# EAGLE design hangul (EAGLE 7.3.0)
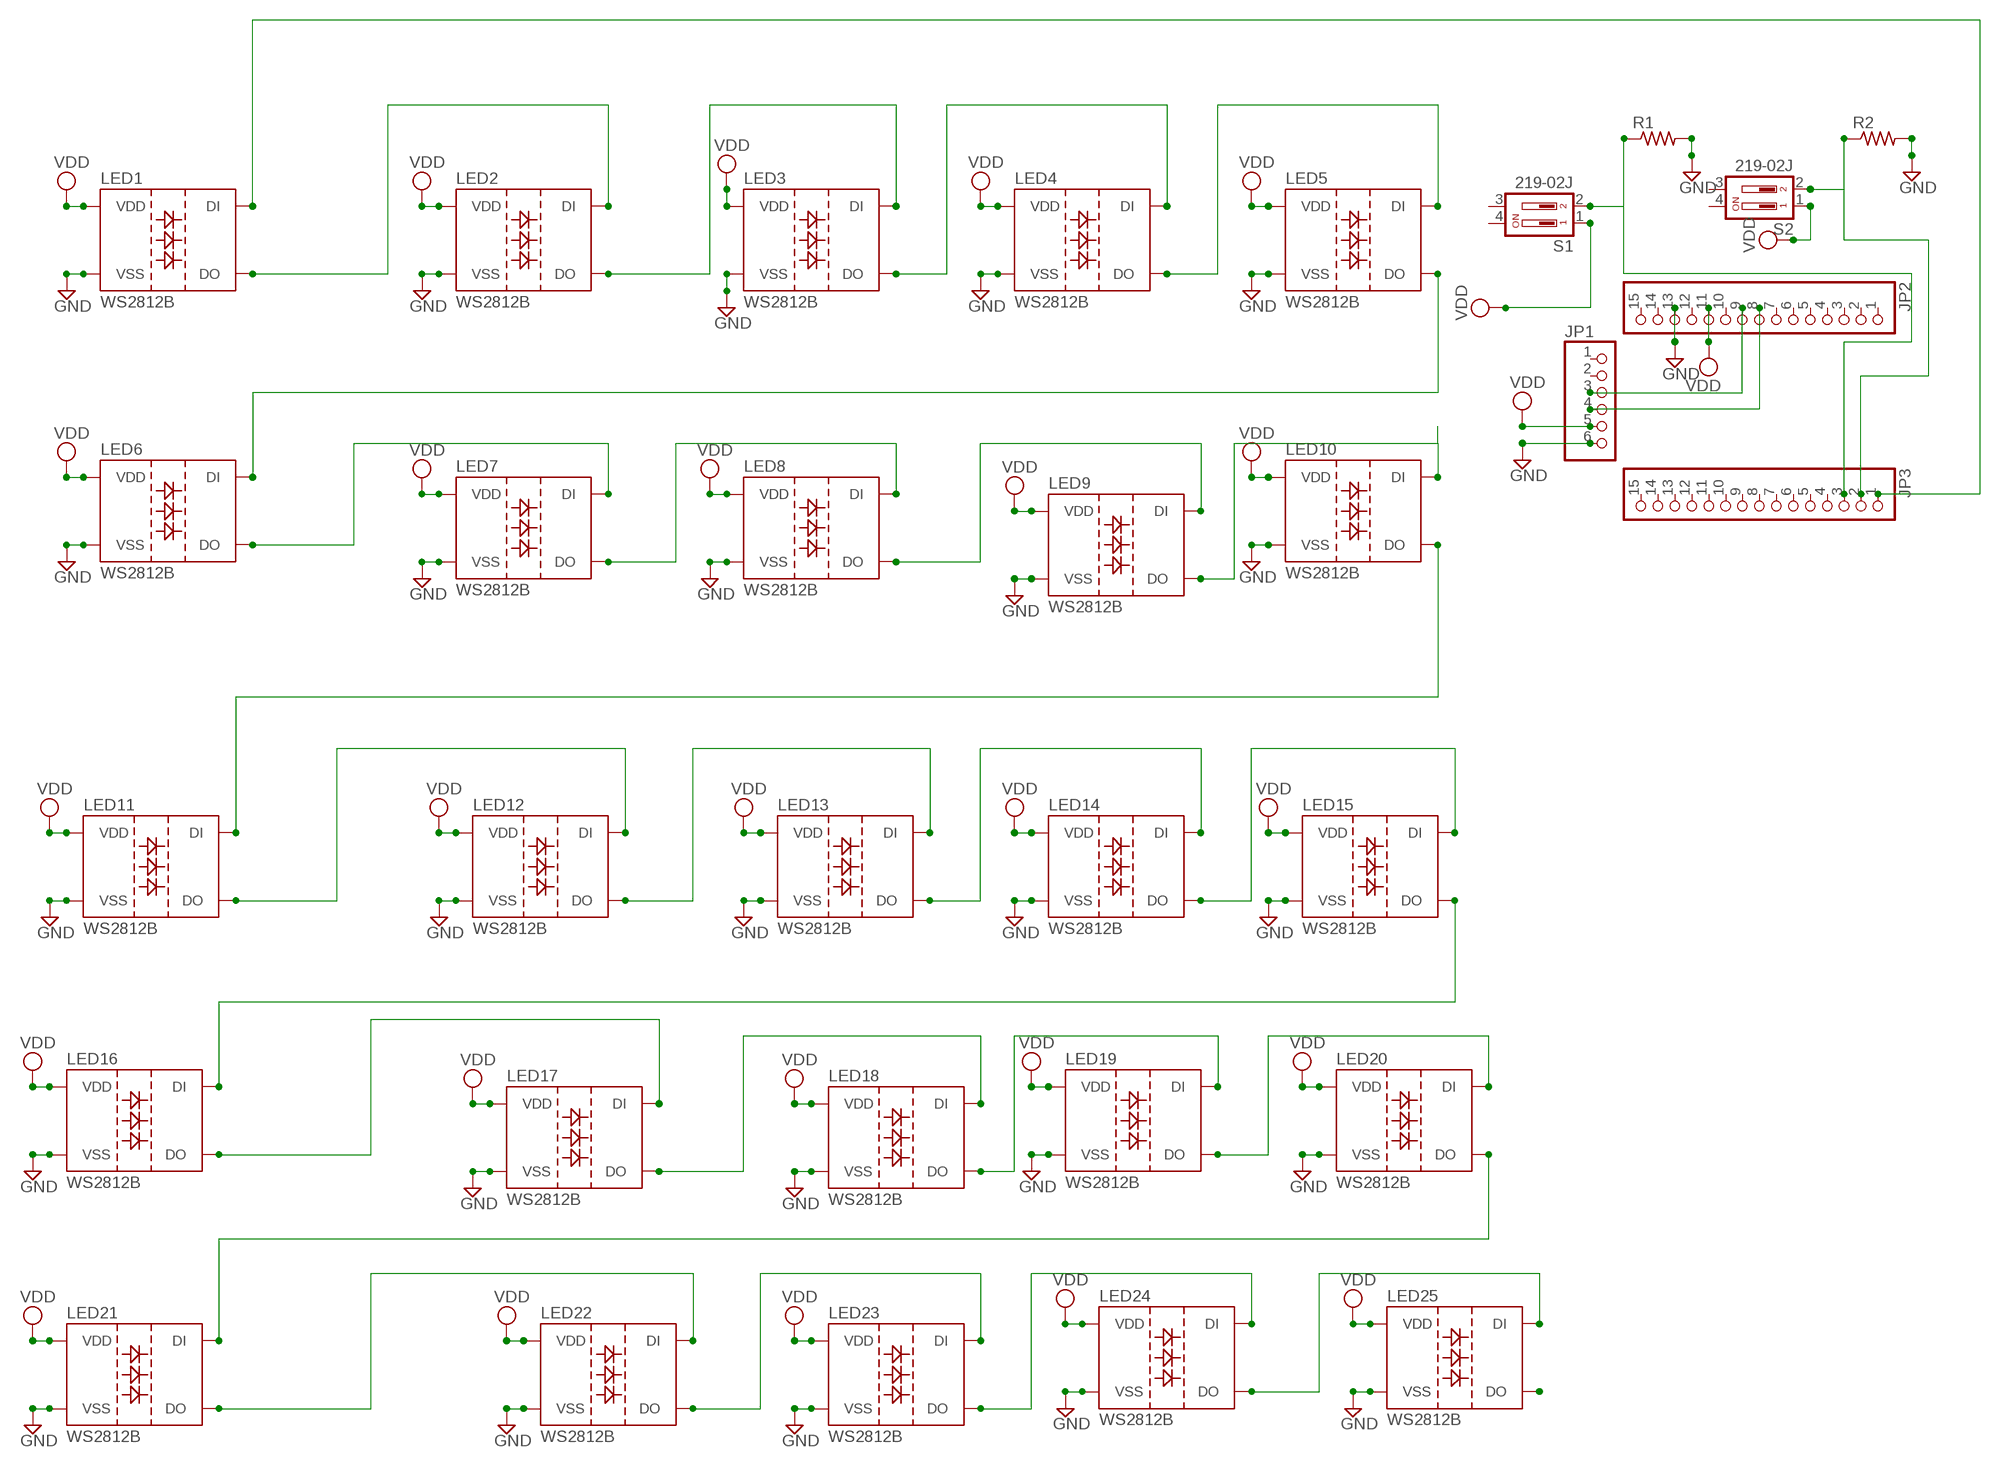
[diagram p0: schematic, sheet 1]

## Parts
JP1  PINHD-1X6  [1X06]
JP2  PINHD-1X15  [1X15]
JP3  PINHD-1X15  [1X15]
LED1  WS2812B  [WS2812B]
LED2  WS2812B  [WS2812B]
LED3  WS2812B  [WS2812B]
LED4  WS2812B  [WS2812B]
LED5  WS2812B  [WS2812B]
LED6  WS2812B  [WS2812B]
LED7  WS2812B  [WS2812B]
LED8  WS2812B  [WS2812B]
LED9  WS2812B  [WS2812B]
LED10  WS2812B  [WS2812B]
LED11  WS2812B  [WS2812B]
LED12  WS2812B  [WS2812B]
LED13  WS2812B  [WS2812B]
LED14  WS2812B  [WS2812B]
LED15  WS2812B  [WS2812B]
LED16  WS2812B  [WS2812B]
LED17  WS2812B  [WS2812B]
LED18  WS2812B  [WS2812B]
LED19  WS2812B  [WS2812B]
LED20  WS2812B  [WS2812B]
LED21  WS2812B  [WS2812B]
LED22  WS2812B  [WS2812B]
LED23  WS2812B  [WS2812B]
LED24  WS2812B  [WS2812B]
LED25  WS2812B  [WS2812B]
R1  R-US_0207/10  [0207/10]
R2  R-US_0207/10  [0207/10]
S1  219-02J  [CTS-219-02J]
S2  219-02J  [CTS-219-02J]

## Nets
GND: JP1.6 JP2.13 LED1.3(VSS) LED2.3(VSS) LED3.3(VSS) LED4.3(VSS) LED5.3(VSS) LED6.3(VSS) LED7.3(VSS) LED8.3(VSS) LED9.3(VSS) LED10.3(VSS) LED11.3(VSS) LED12.3(VSS) LED13.3(VSS) LED14.3(VSS) LED15.3(VSS) LED16.3(VSS) LED17.3(VSS) LED18.3(VSS) LED19.3(VSS) LED20.3(VSS) LED21.3(VSS) LED22.3(VSS) LED23.3(VSS) LED24.3(VSS) LED25.3(VSS) R1.2 R2.2
N$1: JP3.2 R2.1 S2.2
N$2: JP3.3 R1.1 S1.2
N$3: JP3.1 LED1.4(DI)
N$4: LED1.2(DO) LED2.4(DI)
N$7: JP1.3 JP2.9
N$8: LED2.2(DO) LED3.4(DI)
N$12: LED3.2(DO) LED4.4(DI)
N$16: LED4.2(DO) LED5.4(DI)
N$20: LED5.2(DO) LED6.4(DI)
N$21: JP1.4 JP2.8
N$22: LED10.2(DO) LED11.4(DI)
N$26: LED9.2(DO) LED10.4(DI)
N$30: LED8.2(DO) LED9.4(DI)
N$34: LED7.2(DO) LED8.4(DI)
N$38: LED6.2(DO) LED7.4(DI)
N$44: LED11.2(DO) LED12.4(DI)
N$48: LED12.2(DO) LED13.4(DI)
N$52: LED13.2(DO) LED14.4(DI)
N$56: LED14.2(DO) LED15.4(DI)
N$60: LED15.2(DO) LED16.4(DI)
N$62: LED20.2(DO) LED21.4(DI)
N$66: LED19.2(DO) LED20.4(DI)
N$70: LED18.2(DO) LED19.4(DI)
N$74: LED17.2(DO) LED18.4(DI)
N$78: LED16.2(DO) LED17.4(DI)
N$84: LED21.2(DO) LED22.4(DI)
N$88: LED22.2(DO) LED23.4(DI)
N$92: LED23.2(DO) LED24.4(DI)
N$96: LED24.2(DO) LED25.4(DI)
N$100: LED25.2(DO)
VDD: JP1.5 JP2.11 LED1.1(VDD) LED2.1(VDD) LED3.1(VDD) LED4.1(VDD) LED5.1(VDD) LED6.1(VDD) LED7.1(VDD) LED8.1(VDD) LED9.1(VDD) LED10.1(VDD) LED11.1(VDD) LED12.1(VDD) LED13.1(VDD) LED14.1(VDD) LED15.1(VDD) LED16.1(VDD) LED17.1(VDD) LED18.1(VDD) LED19.1(VDD) LED20.1(VDD) LED21.1(VDD) LED22.1(VDD) LED23.1(VDD) LED24.1(VDD) LED25.1(VDD) S1.1 S2.1
Unconnected: JP1.1 JP1.2 JP2.1 JP2.2 JP2.3 JP2.4 JP2.5 JP2.6 JP2.7 JP2.10 JP2.12 JP2.14 JP2.15 JP3.4 JP3.5 JP3.6 JP3.7 JP3.8 JP3.9 JP3.10 JP3.11 JP3.12 JP3.13 JP3.14 JP3.15 S1.3 S1.4 S2.3 S2.4

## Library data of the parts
JP1 = adafruit:PINHD-1X6: PIN HEADER
JP2 JP3 = adafruit:PINHD-1X15: PIN HEADER
LED1-LED25 = WS2812:WS2812B
R1 R2 = adafruit:R-US_: RESISTOR, American symbol
S1 S2 = switch-dil:219-02*: Surface Mount DIP Switch Series 219 SMT CTS Electronic Components Sourc: www.ctscorp.com; OC_FARNELL: unknown; OC_NEWARK: unknown

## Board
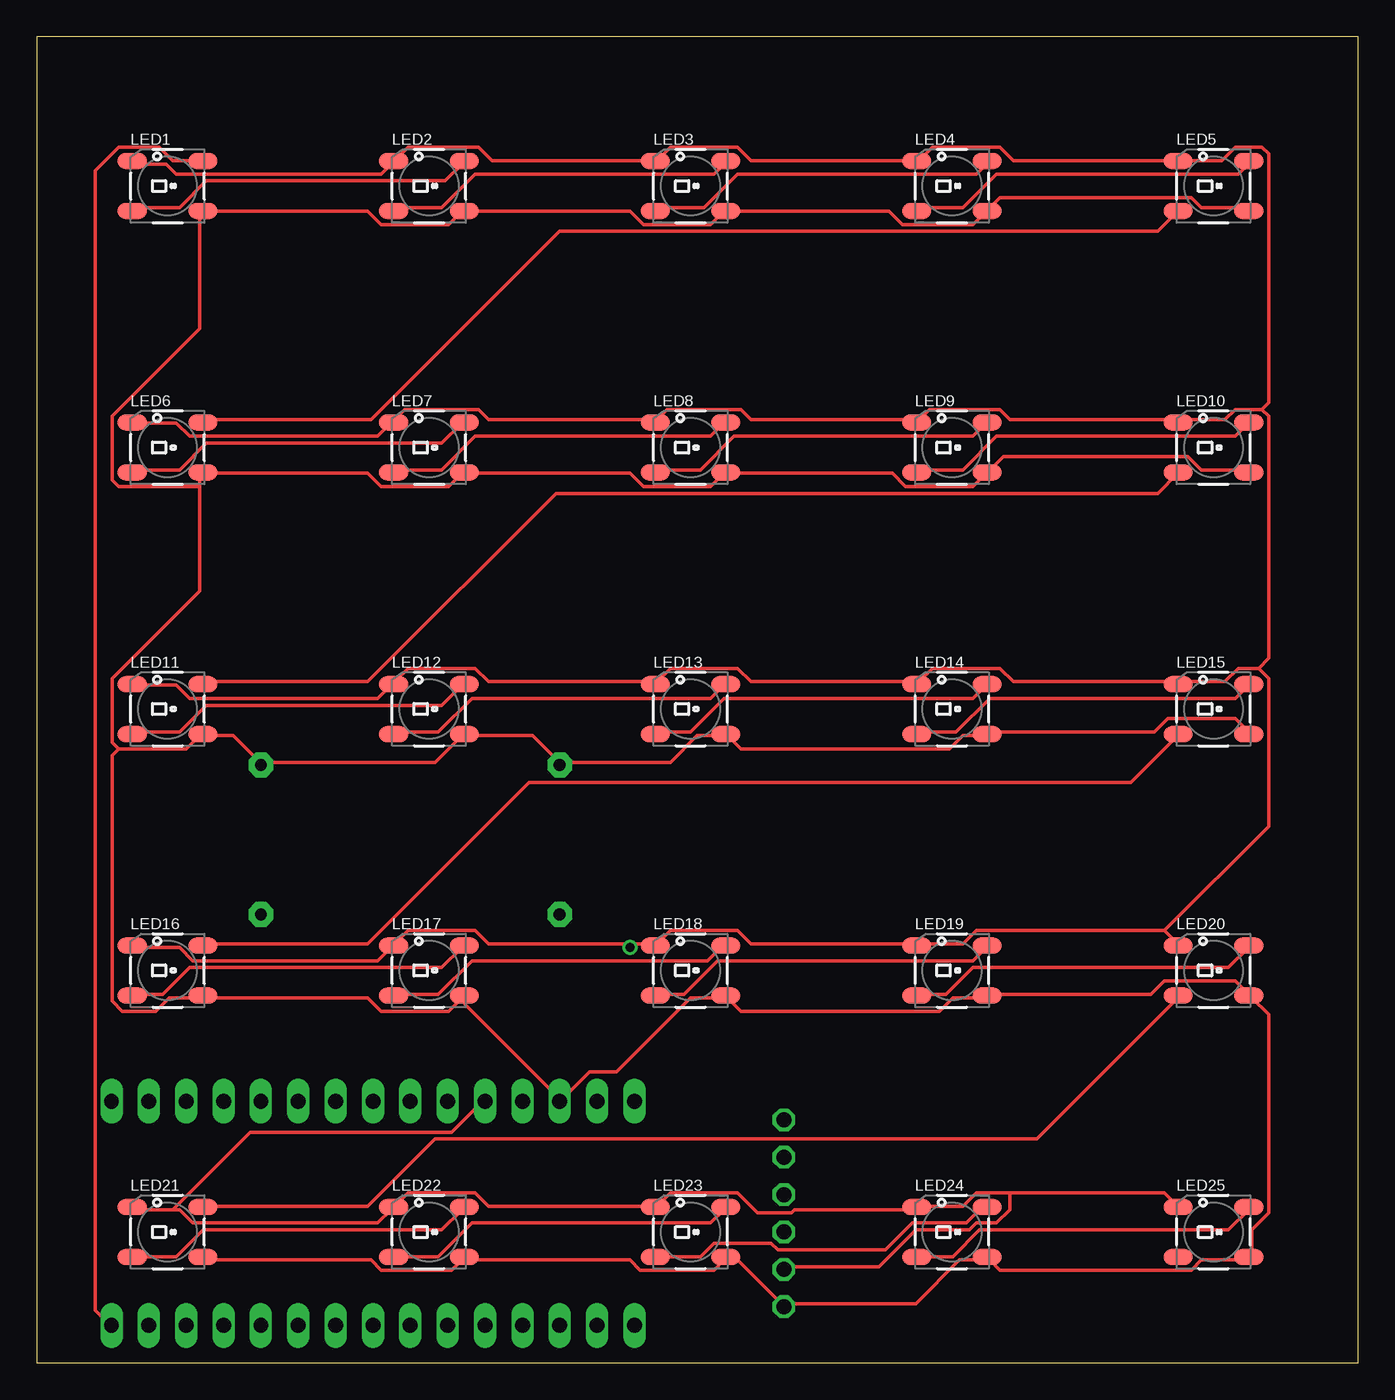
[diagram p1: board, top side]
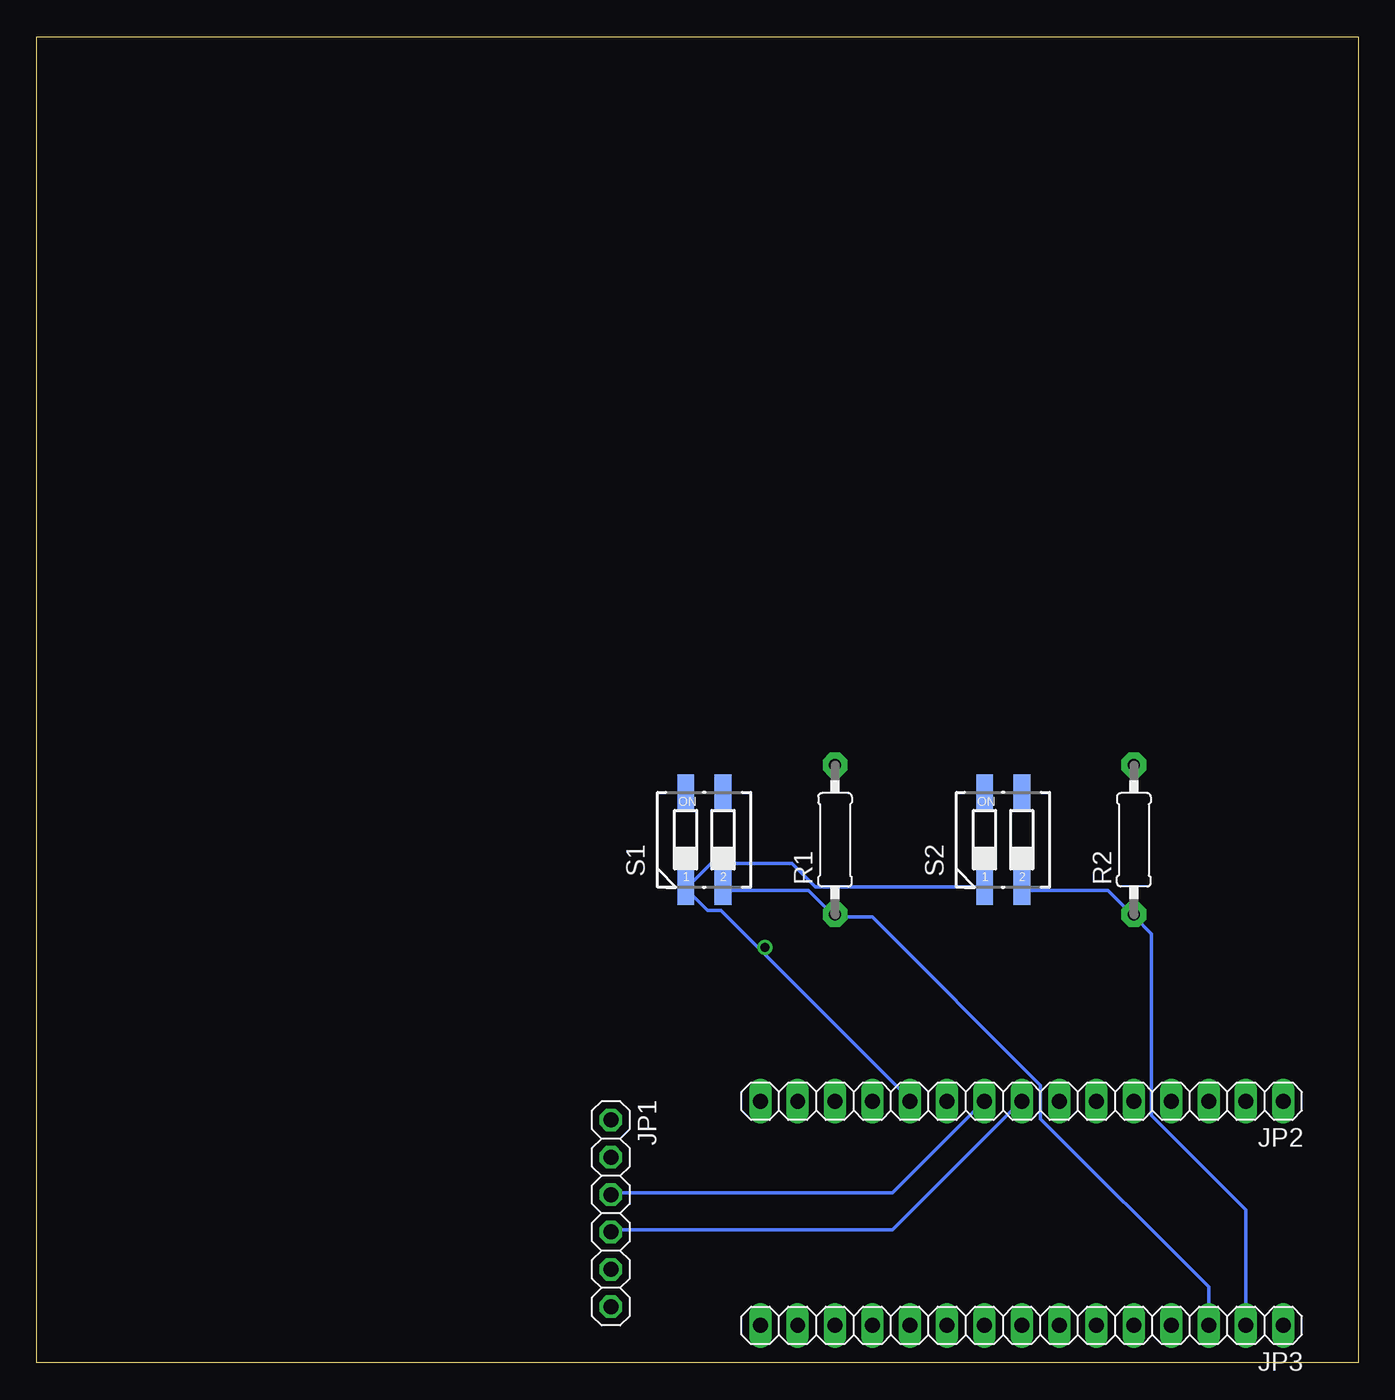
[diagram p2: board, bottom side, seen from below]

Size 89.84 x 90.16 mm. Coordinates in mm from the lower left corner, seen from the top.
Outline: 0,0 89.84,0 89.84,90.16 0,90.16 0,0
Copper layers (1*16): Top 0.035mm / dielectric 1.5mm / Bottom 0.035mm
Design rules "default": minimum track width 10mil, minimum drill 24mil, track to track 8mil, track to pad 8mil, pad to pad 8mil, via to via 8mil, smd to smd 8mil, copper to edge 40mil, drill to drill 8mil, minimum pad ring 10mil, minimum via ring 8mil, stop-mask expansion 4mil, vias tented up to drill 0mil, thermal gap 10mil

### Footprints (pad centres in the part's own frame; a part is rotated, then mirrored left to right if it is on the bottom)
1X06 = drill 1.016 octagon: 1 -6.35,0; 2 -3.81,0; 3 -1.27,0; 4 1.27,0; 5 3.81,0; 6 6.35,0
1X15 = drill 1.016 long: 1 -17.78,0; 2 -15.24,0; 3 -12.7,0; 4 -10.16,0; 5 -7.62,0; 6 -5.08,0; 7 -2.54,0; 8 0,0; 9 2.54,0; 10 5.08,0; 11 7.62,0; 12 10.16,0; 13 12.7,0; 14 15.24,0; 15 17.78,0
WS2812B = smd 2 x 1.1: 1 -2.4,1.7; 2 -2.4,-1.7; 3 2.4,-1.7; 4 2.4,1.7
0207/10 = drill 0.813 pad 1.676 octagon: 1 -5.08,0; 2 5.08,0
CTS-219-02J = smd 1.13 x 2.44: 1 -1.27,-3.215; 2 1.27,-3.215; 3 1.27,3.215; 4 -1.27,3.215

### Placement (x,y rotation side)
JP1  50.8,10.16 270 bottom
JP2  22.86,17.78 180 bottom
JP3  22.86,2.54 180 bottom
LED1  8.89,80.01 0 top
LED2  26.67,80.01 0 top
LED3  44.45,80.01 0 top
LED4  62.23,80.01 0 top
LED5  80.01,80.01 0 top
LED6  8.89,62.23 0 top
LED7  26.67,62.23 0 top
LED8  44.45,62.23 0 top
LED9  62.23,62.23 0 top
LED10  80.01,62.23 0 top
LED11  8.89,44.45 0 top
LED12  26.67,44.45 0 top
LED13  44.45,44.45 0 top
LED14  62.23,44.45 0 top
LED15  80.01,44.45 0 top
LED16  8.89,26.67 0 top
LED17  26.67,26.67 0 top
LED18  44.45,26.67 0 top
LED19  62.23,26.67 0 top
LED20  80.01,26.67 0 top
LED21  8.89,8.89 0 top
LED22  26.67,8.89 0 top
LED23  44.45,8.89 0 top
LED24  62.23,8.89 0 top
LED25  80.01,8.89 0 top
R1  35.56,35.56 90 bottom
R2  15.24,35.56 90 bottom
S1  44.45,35.56 0 bottom
S2  24.13,35.56 0 bottom

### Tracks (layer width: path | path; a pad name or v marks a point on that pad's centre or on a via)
GND
  Top 0.254: LED21.3 11.3,6.98 22.73,6.98 23.42,6.3 28.22,6.3 28.91,6.98 LED22.3 29.13,6.98 40.33,6.98 41.02,6.3 46.05,6.3 46.74,6.98 LED23.3 46.96,6.98 47.65,6.98 50.62,4.01 JP1.6 50.85,4.01 59.77,4.01 62.74,6.98 64.57,6.98 LED24.3 64.8,6.98 65.48,6.3 78.51,6.3 79.2,6.98 82.4,6.98 LED25.3 82.63,7.21 82.63,9.04 83.77,10.18 83.77,23.67 82.63,24.82 LED20.3 82.4,25.04 81.48,25.96 76.68,25.96 75.77,25.04 64.8,25.04 LED19.3 64.57,24.82 62.28,24.82 61.37,23.9 47.88,23.9 46.96,24.82 LED18.3 46.74,24.82 44.45,24.82 39.42,19.79 37.59,19.79 35.76,17.96 JP2.13 35.53,17.96 29.13,24.36 29.13,24.82 LED17.3 28.91,24.82 27.99,23.9 23.42,23.9 22.5,24.82 11.3,24.82 LED16.3 11.07,24.82 9.02,24.82 8.1,23.9 5.82,23.9 5.13,24.59 5.13,41.28 5.59,41.73 | LED5.3 82.4,78.54 79.2,78.54 78.51,79.22 65.48,79.22 64.8,78.54 LED4.3 64.57,78.31 63.65,77.39 58.85,77.39 57.94,78.31 46.96,78.31 LED3.3 46.74,78.31 45.82,77.39 41.25,77.39 40.33,78.31 29.13,78.31 LED2.3 28.91,78.31 27.99,77.39 23.42,77.39 22.5,78.31 11.3,78.31 LED1.3 11.07,78.31 11.07,70.31 5.13,64.36 5.13,60.02 5.59,59.56 11.07,59.56 | LED10.3 82.4,60.71 79.2,60.71 78.28,61.62 65.71,61.62 64.8,60.71 LED9.3 64.57,60.48 63.65,59.56 59.08,59.56 58.17,60.48 46.96,60.48 LED8.3 46.74,60.48 45.82,59.56 41.25,59.56 40.33,60.48 29.13,60.48 LED7.3 28.91,60.48 27.99,59.56 23.42,59.56 22.5,60.48 11.3,60.48 LED6.3 11.07,60.48 11.07,59.56 | LED15.3 82.4,42.88 81.48,43.79 76.91,43.79 76,42.88 64.8,42.88 LED14.3 64.57,42.65 62.97,42.65 62.05,41.73 47.88,41.73 46.96,42.65 LED13.3 46.74,42.65 44.91,42.65 43.08,40.82 35.76,40.82 R1.2 35.53,40.82 33.71,42.65 29.13,42.65 LED12.3 28.91,42.65 27.08,40.82 15.42,40.82 R2.2 15.19,40.82 13.36,42.65 11.3,42.65 LED11.3 11.07,42.65 10.16,41.73 5.59,41.73
  Top 0.254: 11.07,59.56 11.07,52.48 5.13,46.53 5.13,42.19 5.59,41.73
N$1
  Bottom 0.254: S2.2 22.73,32.13 17.02,32.13 15.42,30.53 R2.1 15.19,30.3 14.05,29.16 14.05,16.82 7.64,10.41 7.64,2.64 JP3.2
N$2
  Bottom 0.254: S1.2 43.08,32.13 37.36,32.13 35.76,30.53 R1.1 35.53,30.3 33.02,30.3 21.59,18.87 21.59,16.59 10.16,5.16 JP3.3
N$3
  Top 0.254: LED1.4 11.07,81.74 9.25,81.74 8.33,82.65 5.59,82.65 3.99,81.05 3.99,3.56 4.9,2.64 JP3.1
N$4
  Top 0.254: LED1.2 6.5,78.54 9.7,78.54 11.53,80.37 27.76,80.37 28.91,81.51 LED2.4
N$7
  Bottom 0.254: JP1.3 50.62,11.56 31.65,11.56 25.48,17.73 JP2.9
N$8
  Top 0.254: LED2.2 24.33,78.54 27.53,78.54 29.82,80.82 46.05,80.82 46.74,81.51 LED3.4
N$12
  Top 0.254: LED3.2 42.16,78.54 45.36,78.54 47.65,80.82 63.88,80.82 64.57,81.51 LED4.4
N$16
  Top 0.254: LED4.2 59.99,78.54 62.97,78.54 65.25,80.82 81.71,80.82 82.4,81.51 LED5.4
N$20
  Top 0.254: LED6.4 11.3,64.14 22.73,64.14 35.53,76.94 76.23,76.94 77.6,78.31 LED5.2
N$21
  Bottom 0.254: JP1.4 50.62,9.04 31.65,9.04 22.96,17.73 JP2.8
N$22
  Top 0.254: LED11.4 11.3,46.3 22.5,46.3 35.31,59.11 76.23,59.11 77.6,60.48 LED10.2
N$26
  Top 0.254: LED9.2 59.99,60.71 62.97,60.71 65.25,62.99 81.48,62.99 82.4,63.91 LED10.4
N$30
  Top 0.254: LED8.2 42.16,60.71 45.14,60.71 47.42,62.99 63.65,62.99 64.57,63.91 LED9.4
N$34
  Top 0.254: LED7.2 24.33,60.71 27.53,60.71 29.82,62.99 45.82,62.99 46.74,63.91 LED8.4
N$38
  Top 0.254: LED6.2 6.5,60.71 9.7,60.71 11.53,62.54 27.53,62.54 28.91,63.91 LED7.4
N$44
  Top 0.254: LED11.2 6.5,42.88 9.7,42.88 11.53,44.7 27.53,44.7 28.91,46.08 LED12.4
N$48
  Top 0.254: LED12.2 24.33,42.88 27.3,42.88 29.59,45.16 45.82,45.16 46.74,46.08 LED13.4
N$52
  Top 0.254: LED13.2 42.16,42.88 44.45,42.88 46.74,45.16 63.65,45.16 64.57,46.08 LED14.4
N$56
  Top 0.254: LED14.2 59.99,42.88 62.51,42.88 64.8,45.16 81.48,45.16 82.4,46.08 LED15.4
N$60
  Top 0.254: LED16.4 11.3,28.47 22.5,28.47 33.48,39.45 74.4,39.45 77.6,42.65 LED15.2
N$62
  Top 0.254: LED21.4 11.3,10.64 22.5,10.64 27.08,15.21 68,15.21 77.6,24.82 LED20.2
N$66
  Top 0.254: LED19.2 59.99,25.04 61.82,25.04 63.65,26.87 81.03,26.87 82.4,28.25 LED20.4
N$70
  Top 0.254: LED18.2 42.16,25.04 43.99,25.04 46.28,27.33 63.65,27.33 64.57,28.25 LED19.4
N$74
  Top 0.254: LED17.2 24.33,25.04 27.3,25.04 29.59,27.33 45.59,27.33 46.74,28.47 LED18.4
N$78
  Top 0.254: LED16.2 6.5,25.04 8.56,25.04 10.39,26.87 27.53,26.87 28.91,28.25 LED17.4
N$84
  Top 0.254: LED21.2 6.5,7.21 9.47,7.21 11.3,9.04 27.53,9.04 28.91,10.41 LED22.4
N$88
  Top 0.254: LED22.2 24.33,7.21 27.3,7.21 29.59,9.5 45.82,9.5 46.74,10.41 LED23.4
N$92
  Top 0.254: LED23.2 42.16,7.21 45.14,7.21 46.05,8.13 49.94,8.13 50.39,7.67 57.71,7.67 59.54,9.5 63.2,9.5 64.11,10.41 64.57,10.41 LED24.4
N$96
  Top 0.254: LED24.2 59.99,7.21 62.28,7.21 64.11,9.04 81.03,9.04 82.4,10.41 LED25.4
VDD  (via drill 0.61)
  Top 0.254: LED1.1 6.5,81.51 8.79,81.51 9.47,80.82 23.42,80.82 24.11,81.51 LED2.1 24.33,81.74 25.25,82.65 30.05,82.65 30.96,81.74 41.93,81.74 LED3.1 42.16,81.74 43.08,82.65 47.65,82.65 48.56,81.74 59.77,81.74 LED4.1 59.99,81.74 60.91,82.65 65.48,82.65 66.4,81.74 77.6,81.74 LED5.1 77.83,81.74 80.57,81.74 81.48,82.65 83.31,82.65 83.77,82.19 83.77,65.28 83.31,64.82 | LED6.1 6.5,63.91 9.47,63.91 10.39,62.99 23.19,62.99 24.11,63.91 LED7.1 24.33,64.14 25.02,64.82 30.05,64.82 30.73,64.14 41.93,64.14 LED8.1 42.16,64.14 42.85,64.82 47.88,64.82 48.56,64.14 59.77,64.14 LED9.1 59.99,64.14 60.68,64.82 65.48,64.82 66.17,64.14 77.6,64.14 LED10.1 77.83,64.14 80.8,64.14 81.48,64.82 83.31,64.82 | LED11.1 6.5,46.08 9.47,46.08 10.39,45.16 23.19,45.16 24.11,46.08 LED12.1 24.33,46.3 25.25,47.22 29.82,47.22 30.73,46.3 41.93,46.3 LED13.1 42.16,46.3 43.08,47.22 47.65,47.22 48.56,46.3 59.77,46.3 LED14.1 59.99,46.3 60.91,47.22 65.48,47.22 66.4,46.3 77.6,46.3 LED15.1 77.83,46.3 80.8,46.3 81.71,47.22 83.08,47.22 | 76.68,29.39 63.88,29.39 62.97,28.47 59.99,28.47 LED19.1 59.77,28.47 48.56,28.47 47.65,29.39 43.08,29.39 42.16,28.47 LED18.1 41.93,28.47 40.33,28.47 | 76.68,29.39 77.6,28.47 LED20.1 | LED16.1 6.5,28.25 9.7,28.25 10.62,27.33 23.19,27.33 24.11,28.25 LED17.1 24.33,28.47 25.25,29.39 29.82,29.39 30.73,28.47 40.33,28.47 | 66.17,11.56 76.68,11.56 77.6,10.64 LED25.1 | 66.17,11.56 63.88,11.56 62.97,10.64 59.99,10.64 LED24.1 59.77,10.41 51.54,10.41 51.31,10.18 49.02,10.18 47.65,11.56 43.08,11.56 42.16,10.64 LED23.1 41.93,10.64 30.73,10.64 29.82,11.56 25.25,11.56 24.33,10.64 LED22.1 24.11,10.41 23.19,9.5 10.62,9.5 9.7,10.41 9.25,10.41
  Top 0.254: 66.17,11.56 66.17,10.41 65.25,9.5 63.88,9.5 63.42,9.04 59.77,9.04 57.25,6.53 50.85,6.53 JP1.5 | 9.25,10.41 6.5,10.41 LED21.1 | 9.25,10.41 14.5,15.67 28.22,15.67 30.28,17.73 JP2.11 | v40.33,28.25 40.33,28.47 | 83.08,47.22 83.77,46.53 83.77,36.47 76.68,29.39 | 83.31,64.82 83.77,64.36 83.77,47.9 83.08,47.22
  Bottom 0.254: S2.1 25.48,32.36 36.91,32.36 38.51,33.96 43.99,33.96 45.59,32.36 S1.1 45.59,32.13 44.22,30.76 43.31,30.76 40.56,28.02 | 40.56,28.02 30.5,17.96 JP2.11 | 40.56,28.02 v40.33,28.25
